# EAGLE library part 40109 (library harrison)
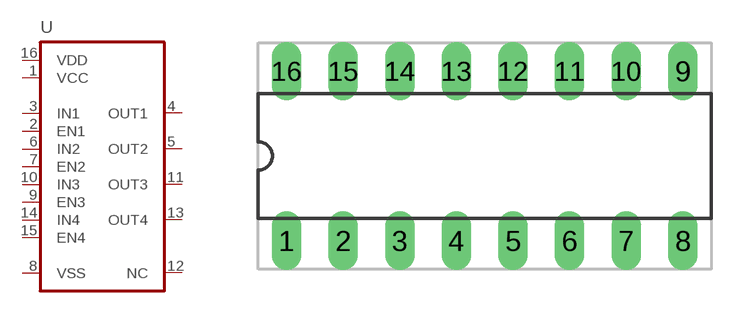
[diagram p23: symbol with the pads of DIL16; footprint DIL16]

Designator prefix U

## 40109  [DIL16]
1  VCC  pwr
2  EN1  in
3  IN1  in
4  OUT1  out
5  OUT2  out
6  IN2  in
7  EN2  in
8  VSS  pwr
9  EN3  in
10  IN3  in
11  OUT3  out
12  NC  nc
13  OUT4  out
14  IN4  in
15  EN4  in
16  VDD  pwr

## Footprint DIL16 (pad centres in mm)
drill 0.813 long: 1 -8.89,-3.81; 2 -6.35,-3.81; 3 -3.81,-3.81; 4 -1.27,-3.81; 5 1.27,-3.81; 6 3.81,-3.81; 7 6.35,-3.81; 8 8.89,-3.81; 9 8.89,3.81; 10 6.35,3.81; 11 3.81,3.81; 12 1.27,3.81; 13 -1.27,3.81; 14 -3.81,3.81; 15 -6.35,3.81; 16 -8.89,3.81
